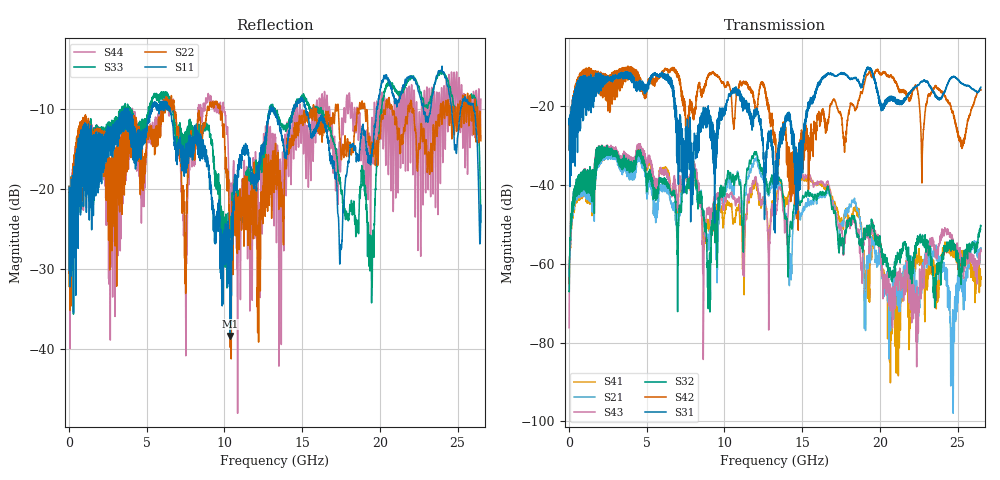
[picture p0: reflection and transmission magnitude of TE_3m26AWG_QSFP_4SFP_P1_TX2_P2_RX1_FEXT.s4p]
!Agilent Technologies,N5222A,MY51421691,A.10.00.00
!Agilent N5222A: A.10.00.00
!Date: Friday, January 30, 2015 12:37:23
!Correction: S11(Full 4 Port(1,2,3,4))
!S12(Full 4 Port(1,2,3,4))
!S13(Full 4 Port(1,2,3,4))
!S14(Full 4 Port(1,2,3,4))
!S21(Full 4 Port(1,2,3,4))
!S22(Full 4 Port(1,2,3,4))
!S23(Full 4 Port(1,2,3,4))
!S24(Full 4 Port(1,2,3,4))
!S31(Full 4 Port(1,2,3,4))
!S32(Full 4 Port(1,2,3,4))
!S33(Full 4 Port(1,2,3,4))
!S34(Full 4 Port(1,2,3,4))
!S41(Full 4 Port(1,2,3,4))
!S42(Full 4 Port(1,2,3,4))
!S43(Full 4 Port(1,2,3,4))
!S44(Full 4 Port(1,2,3,4))
!S4P File: Measurements: <S11,S12,S13,S14>,
!<S21,S22,S23,S24>,
!<S31,S32,S33,S34>,
!<S41,S42,S43,S44>:
# Hz S  dB  R 50.0
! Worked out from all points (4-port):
!   2650 points, 10 MHz to 26.5 GHz, reference 50 ohm
!   strongest paths, dB at 10 MHz, 6.63 GHz, 13.26 GHz, 19.88 GHz, 26.5 GHz:
!     S31: -24.7, -15.5, -42.5, -17.3, -15.3
!     S42: -24.8, -11.0, -27.4, -11.0, -16.0
!     S32: -67.0, -42.3, -40.4, -55.0, -50.4
!     S43: -76.3, -42.0, -46.6, -53.4, -56.8
!     S21: -61.5, -45.2, -41.3, -58.0, -56.0
!     S41: -60.7, -42.2, -44.3, -53.2, -63.9
!   lowest |S11| = -38.4 dB at 10.38 GHz (marker M1), VSWR 1.02, Z = 49 + j0.647 ohm
!   |S11| at or under -10 dB: start of sweep to 3.58 GHz; 6.486 GHz to 12.98 GHz (6.492 GHz wide, 66.7 % of centre); 15.24 GHz to 19.79 GHz (4.547 GHz wide, 26 % of centre)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
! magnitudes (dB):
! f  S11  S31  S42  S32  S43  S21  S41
! 10 MHz  -19.8  -24.7  -24.8  -67.0  -76.3  -61.5  -60.7
! 2.04 GHz  -13.5  -11.8  -11.4  -33.8  -33.2  -34.5  -34.4
! 9.01 GHz  -18.3  -23.6  -11.8  -63.2  -45.7  -53.3  -48.8
! 10.38 GHz  -38.4  -17.6  -15.8  -37.0  -42.2  -38.7  -44.9
! 13.3 GHz  -11.1  -36.3  -28.9  -39.1  -47.5  -40.7  -44.1
! 24.66 GHz  -11.1  -12.8  -21.9  -55.0  -53.5  -77.7  -56.7
! 26.5 GHz  -22.1  -15.3  -16.0  -50.4  -56.8  -56.0  -63.9
